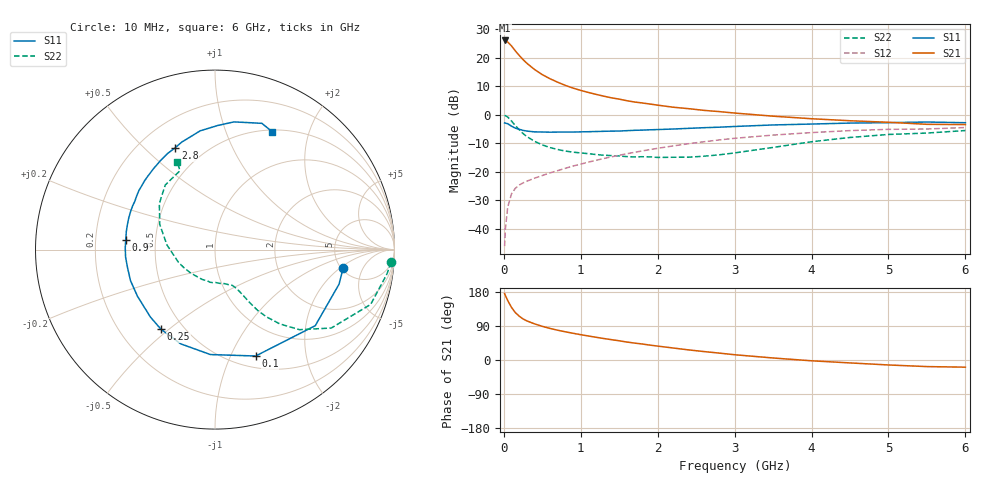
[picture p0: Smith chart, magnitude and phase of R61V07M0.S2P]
! SIEMENS Small Signal Semiconductors
! BFR193
! Si NPN RF Bipolar Junction Transistor in SOT23
! VCE = 1 V  IC = 7 mA
! Common Emitter S-Parameters:  May  1996
# GHz  S  MA  R  50
!  f  S11  S21  S12  S22
! GHz  MAG  ANG  MAG  ANG  MAG  ANG  MAG  ANG
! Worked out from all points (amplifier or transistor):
!   36 points, 10 MHz to 6 GHz, reference 50 ohm
!   highest |S21| = 26.1 dB at 10 MHz (marker M1)
!   |S21| within 3 dB of that: start of sweep to 130.5 MHz
!   unconditionally stable (mu >= 1): 781 MHz to 2.193 GHz
!   at 250 MHz: K = 0.54, MSG = 21.6 dB, |S12| = -23.8 dB
!   at 1.4 GHz: K = 1.06, MAG = 8.8 dB, |S12| = -14.7 dB
!   at 6 GHz: K = 0.98, MSG = 0.5 dB, |S12| = -4.4 dB
!   S11 on the Smith chart (normalised r, x): 10 MHz: 5.24, -2.20; 100 MHz: 0.63, -1.25; 250 MHz: 0.38, -0.47; 900 MHz: 0.33, +0.05; 2.8 GHz: 0.35, +0.63; 6 GHz: 0.52, +1.47
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0.01  0.7219 -8.0  20.19 175.3  0.005 86.3  0.9841 -4.1
0.02  0.7174 -15.6  20.05 170.2  0.01 81.2  0.9674 -8.1
0.05  0.7012 -37.2  18.92 157.0  0.0241 72.5  0.9194 -19.4
0.1  0.6346 -69.1  16.17 138.6  0.0414 60.9  0.7814 -34.0
0.15  0.5853 -92.5  13.21 125.0  0.0518 53.8  0.6482 -43.5
0.2  0.5588 -110.0  11.04 115.7  0.0589 50.2  0.5493 -48.9
0.25  0.5363 -124.1  9.319 108.3  0.0643 48.5  0.4713 -52.6
0.3  0.5203 -133.8  8.02 103.1  0.0689 48.6  0.4153 -54.9
0.4  0.5041 -149.0  6.24 95.3  0.0779 49.2  0.3445 -57.1
0.5  0.5016 -159.9  5.08 88.8  0.0866 50.7  0.2982 -58.4
0.6  0.4976 -168.4  4.308 83.3  0.0963 52.4  0.2677 -59.8
0.7  0.5 -175.3  3.742 78.6  0.1055 54.0  0.2475 -61.1
0.9  0.5004 173.6  2.951 70.5  0.127 55.5  0.2224 -64.0
1.1  0.5077 163.8  2.474 63.3  0.1488 56.6  0.2091 -69.0
1.3  0.5161 155.6  2.128 56.7  0.1722 56.6  0.1963 -74.7
1.6  0.5294 145.5  1.773 47.4  0.2088 55.5  0.1858 -85.9
2.2  0.5655 127.5  1.365 31.7  0.2861 50.4  0.1811 -113.6
2.8  0.6093 111.3  1.143 18.2  0.3641 42.6  0.1997 -149.3
3.5  0.6669 97.1  0.95 5.3  0.4428 31.7  0.2692 174.4
4.5  0.7191 81.6  0.79 -7.7  0.5307 16.3  0.4025 140.4
5.5  0.7504 69.6  0.684 -17.4  0.5661 1.1  0.4806 114.0
6  0.7297 64.0  0.677 -18.9  0.6004 -3.4  0.5321 113.2
